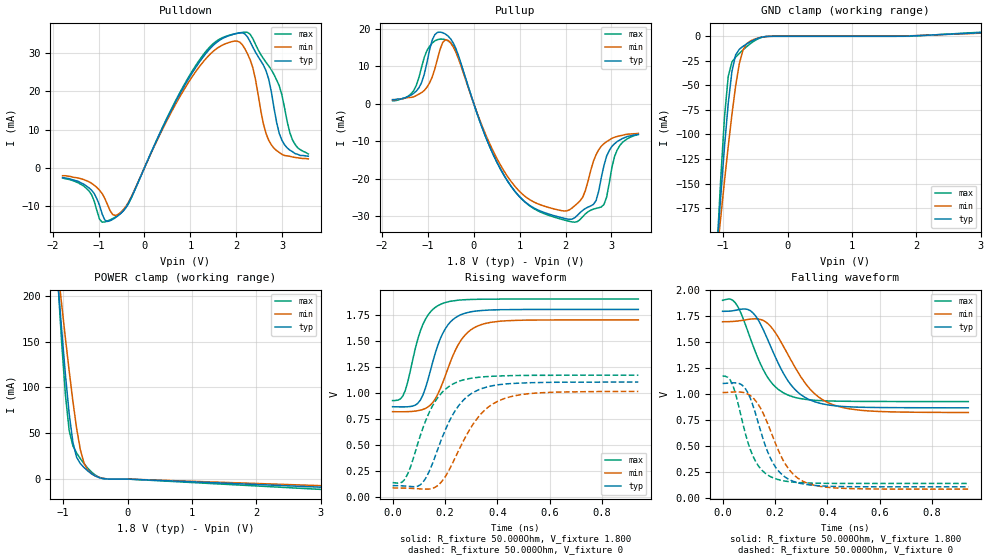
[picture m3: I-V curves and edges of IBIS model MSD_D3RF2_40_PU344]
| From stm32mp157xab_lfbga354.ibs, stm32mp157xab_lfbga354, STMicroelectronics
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[Model] MSD_D3RF2_40_PU344
Model_type   I/O
C_comp 2.316pF   2.235pF   2.435pF
Vinh = 1.150V
Vinl = 650.000mV
Vmeas = 900.000mV
Vref = 900.000mV
[Model Spec]
Vinh   1.150V   1.100V   1.200V
Vinl   650.000mV   600.000mV   700.000mV
Vmeas   900.000mV   850.000mV   950.000mV
Vref   900.000mV   850.000mV   950.000mV
[Temperature Range]   25.000   125.000   -40.000
[Voltage Range]   1.800V   1.700V   1.900V
[GND Clamp Reference]   0.00V   0.00V   0.00V
[Pulldown Reference]   0.00V   0.00V   0.00V
[POWER Clamp Reference]   1.800V   1.700V   1.900V
[Pullup Reference]   1.800V   1.700V   1.900V
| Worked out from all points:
|   slope of the pulldown table from 0 to 0.27 V, typ, clamps not added: 37.2 ohm
|   slope of the pullup table from 0 to 0.27 V, typ, clamps not added: 29.4 ohm
|   GND clamp passes 1 mA (typ) near -0.41 V on its own axis
|   POWER clamp passes 1 mA (typ) near -0.41 V on its own axis
|   rising waveform, R_fixture 50.000Ohm, V_fixture 1.800: 20-80 % time 74.7ps typ, 92.7ps min, 65.8ps max; typ from 0.865 V to 1.8 V
|   rising waveform, R_fixture 50.000Ohm, V_fixture 0: 20-80 % time 111ps typ, 131ps min, 99.4ps max; typ from 0.106 V to 1.1 V
|   falling waveform, R_fixture 50.000Ohm, V_fixture 1.800: 20-80 % time 116ps typ, 136ps min, 101ps max; typ from 1.8 V to 0.868 V
|   falling waveform, R_fixture 50.000Ohm, V_fixture 0: 20-80 % time 85.7ps typ, 103ps min, 74.2ps max; typ from 1.1 V to 0.106 V
[GND Clamp]
-1.785V   -901.1mA   -688.6mA   -1.21A
-1.094V   -214.7mA   -220.8mA   -215.3mA
-1.036V   -161.7mA   -183.5mA   -143.3mA
-978.8mV  -112.2mA   -147.2mA   -81.99mA
-921.2mV  -68.46mA   -112.3mA   -40.92mA
-863.6mV  -35.71mA   -79.59mA   -26.13mA
-806.1mV  -18.97mA   -50.59mA   -21.23mA
-748.5mV  -13.2mA    -27.78mA   -17.42mA
-690.9mV  -10.2mA    -13.78mA   -13.86mA
-575.8mV  -5.513mA   -4.723mA   -7.459mA
-287.9mV  -68.99uA   -116uA     -52.99uA
3.57V     5.268mA    4.537mA    6.293mA
[Power Clamp]
-1.77V    882.6mA    689.9mA    1.159A
-1.079V   212.4mA    226.5mA    212.1mA
-1.021V   160.9mA    189.3mA    146.7mA
-963.6mV  112.9mA    152.9mA    90.9mA
-906.1mV  71.15mA    117.8mA    52.89mA
-848.5mV  40.01mA    84.77mA    36.16mA
-790.9mV  23.78mA    55.42mA    28.47mA
-733.3mV  16.97mA    32.21mA    22.3mA
-675.8mV  12.59mA    17.37mA    16.79mA
-618.2mV  8.95mA     9.729mA    11.92mA
-503mV    3.412mA    3.511mA    4.443mA
3.585V    -10.57mA   -8.572mA   -13.43mA
[Pulldown]
-1.785V   -2.6mA     -2.1mA     -2.7mA
-1.209V   -5.3mA     -3.7mA     -6.1mA
-921.2mV  -12.19mA   -6.8mA     -14.29mA
-575.8mV  -12.6mA    -12.25mA   -12.47mA
1.152V    26.93mA    25.79mA    27.43mA
2.073V    35.36mA    32.95mA    35.37mA
2.361V    31.62mA    26.21mA    33.86mA
2.591V    26.91mA    11.5mA     28.62mA
2.764V    19.9mA     6mA        25.7mA
2.994V    7.2mA      3.5mA      19.1mA
3.224V    4.2mA      2.8mA      7.3mA
3.57V     3mA        2.3mA      3.6mA
[Pullup]
-1.77V    1.1mA      1.074mA    800uA
-1.309V   2.8mA      1.847mA    3.516mA
-1.079V   7.9mA      3.542mA    12.43mA
-848.5mV  18.49mA    9.346mA    16.82mA
-618.2mV  18.63mA    17.11mA    17.12mA
-387.9mV  14.68mA    13.71mA    14.14mA
763.6mV   -21.21mA   -19.96mA   -21.19mA
2.145V    -30.84mA   -27.84mA   -31.6mA
2.606V    -26.91mA   -15.4mA    -28.18mA
2.779V    -19.7mA    -11.34mA   -27.59mA
3.124V    -10.1mA    -8.753mA   -12.36mA
3.585V    -8.2mA     -7.926mA   -8.2mA
[Ramp]
R_load=50.000Ohm
dV/dt_r   578.490mV/94.000ps  542.043mV/113.000ps  600.450mV/83.500ps
dV/dt_f   578.490mV/101.500ps  542.043mV/120.500ps  600.450mV/88.000ps
[Rising waveform]
R_fixture=50.000Ohm
V_fixture=1.800
V_fixture_min=1.700
V_fixture_max=1.900
0s        865.1mV    817.3mV    924.2mV
29ps      863.4mV    816.4mV    937.9mV
48ps      863.5mV    816.8mV    1.018V
106ps     928.4mV    831.7mV    1.593V
125ps     1.04V      847.9mV    1.704V
154ps     1.301V     907.7mV    1.801V
192ps     1.572V     1.1V       1.859V
259ps     1.748V     1.496V     1.891V
336ps     1.789V     1.652V     1.898V
938ps     1.8V       1.7V       1.9V
[Rising waveform]
R_fixture=50.000Ohm
V_fixture=0
0s        106.3mV    83.7mV     135.3mV
48ps      102.5mV    82.12mV    172.1mV
115ps     136.4mV    73.43mV    654.2mV
144ps     266.8mV    74.64mV    831.7mV
183ps     527.6mV    132.1mV    984.9mV
240ps     830.9mV    380.3mV    1.095V
288ps     968.5mV    617.6mV    1.133V
336ps     1.036V     791.5mV    1.15V
432ps     1.084V     948.3mV    1.163V
938ps     1.102V     1.012V     1.168V
[Falling waveform]
R_fixture=50.000Ohm
V_fixture=1.800
V_fixture_min=1.700
V_fixture_max=1.900
0s        1.799V     1.698V     1.905V
48ps      1.808V     1.703V     1.883V
68ps      1.818V     1.709V     1.794V
115ps     1.786V     1.726V     1.476V
173ps     1.522V     1.68V      1.158V
250ps     1.127V     1.379V     991.1mV
336ps     942.3mV    1.042V     944.2mV
441ps     884.8mV    882mV      932.2mV
595ps     871mV      833.1mV    929.3mV
938ps     867.9mV    822.9mV    928.2mV
[Falling waveform]
R_fixture=50.000Ohm
V_fixture=0
0s        1.103V     1.014V     1.174V
39ps      1.109V     1.02V      1.086V
87ps      1.053V     1.011V     620.1mV
106ps     959.7mV    986.3mV    464.4mV
135ps     733.7mV    905.9mV    314.4mV
163ps     504.7mV    771mV      236.9mV
192ps     337.1mV    588.6mV    193.8mV
259ps     170.3mV    257.3mV    154mV
345ps     120.8mV    124.5mV    141.5mV
938ps     105.8mV    83.43mV    138.3mV
